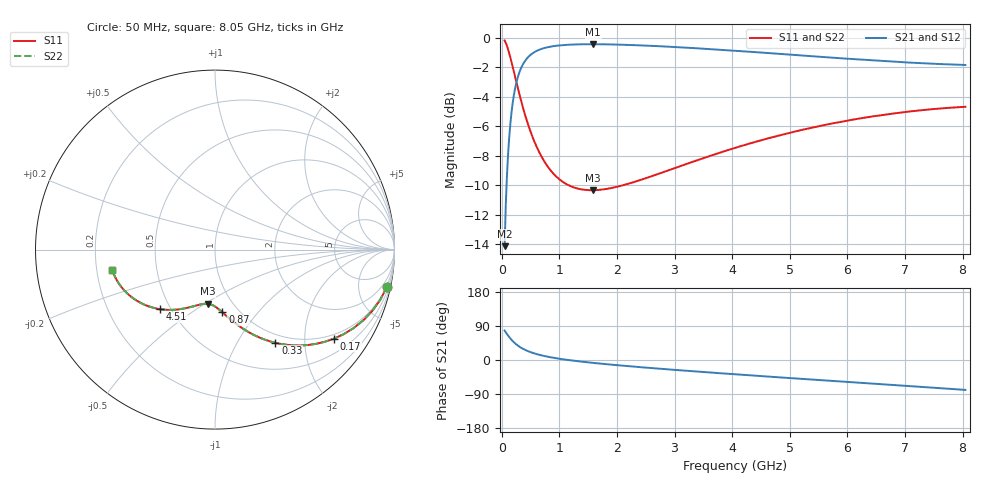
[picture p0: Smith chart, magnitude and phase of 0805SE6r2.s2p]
! AVX Thin Film Operation		Date: August 2001
! Description: Accu-P® Series, Thin Film, SMD, RF Capacitor
! Part Number: 0801J6R2BBT
! 50 MHz  -  8.05 GHz
! Serial Measurements
# mhz S db R 50
!	S11		S21		S12		S22
!	dB	Phase	dB	Phase	dB	Phase	dB	Phase
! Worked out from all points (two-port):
!   401 points, 50 MHz to 8.05 GHz, reference 50 ohm
!   highest |S21| = -0.43 dB at 1.59 GHz (marker M1); lowest = -14.1 dB at 50 MHz (marker M2)
!   |S21| within 3 dB of the highest: 232.5 MHz to end of sweep
!   lowest |S11| = -10.3 dB at 1.59 GHz (marker M3), VSWR 1.88, Z = 38.7 - j25.7 ohm
!   |S11| at or under -10 dB: 1.166 GHz to 2.097 GHz (930.8 MHz wide, 57 % of centre)
!   |S22| runs from -10.3 to -0.2 dB; largest |S21 - S12| = 0
!   S11 on the Smith chart (normalised r, x): 50 MHz: 0.88, -9.31; 170 MHz: 0.87, -2.77; 330 MHz: 0.87, -1.46; 870 MHz: 0.84, -0.67; 4.51 GHz: 0.44, -0.37; 8.05 GHz: 0.26, -0.09
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50  -0.17 -12.2  -14.12 77.8  -14.12 77.8  -0.17 -12.2
90  -0.53 -21.3  -9.40 68.7  -9.40 68.7  -0.53 -21.3
110  -0.77 -25.5  -7.91 64.5  -7.91 64.5  -0.77 -25.5
130  -1.04 -29.5  -6.74 60.5  -6.74 60.5  -1.03 -29.5
170  -1.63 -36.7  -5.05 53.2  -5.05 53.2  -1.63 -36.7
230  -2.60 -45.8  -3.47 44.2  -3.47 44.2  -2.60 -45.8
270  -3.24 -50.8  -2.79 39.2  -2.79 39.2  -3.24 -50.8
330  -4.17 -57.0  -2.10 32.9  -2.10 32.9  -4.17 -57.0
430  -5.54 -65.0  -1.43 25.0  -1.43 25.0  -5.54 -65.0
550  -6.87 -71.8  -1.00 18.1  -1.00 18.1  -6.87 -71.8
690  -8.04 -77.7  -0.74 12.3  -0.74 12.3  -8.04 -77.7
870  -9.08 -83.3  -0.58 6.6  -0.58 6.6  -9.08 -83.3
1110  -9.88 -89.0  -0.47 0.9  -0.47 0.9  -9.88 -89.1
1390  -10.27 -94.3  -0.43 -4.4  -0.43 -4.4  -10.27 -94.3
1590  -10.33 -97.6  -0.43 -7.7  -0.43 -7.7  -10.33 -97.6
2110  -9.99 -105.0  -0.46 -15.1  -0.46 -15.1  -9.99 -105.0
2730  -9.21 -112.7  -0.56 -22.9  -0.56 -22.9  -9.21 -112.8
4050  -7.46 -127.6  -0.87 -37.7  -0.87 -37.7  -7.46 -127.6
4510  -6.93 -132.4  -0.99 -42.6  -0.99 -42.6  -6.93 -132.5
5390  -6.08 -141.5  -1.24 -51.7  -1.24 -51.7  -6.08 -141.6
6730  -5.16 -155.1  -1.59 -65.3  -1.59 -65.3  -5.16 -155.2
8050  -4.67 -168.7  -1.83 -78.9  -1.83 -78.9  -4.67 -168.7
